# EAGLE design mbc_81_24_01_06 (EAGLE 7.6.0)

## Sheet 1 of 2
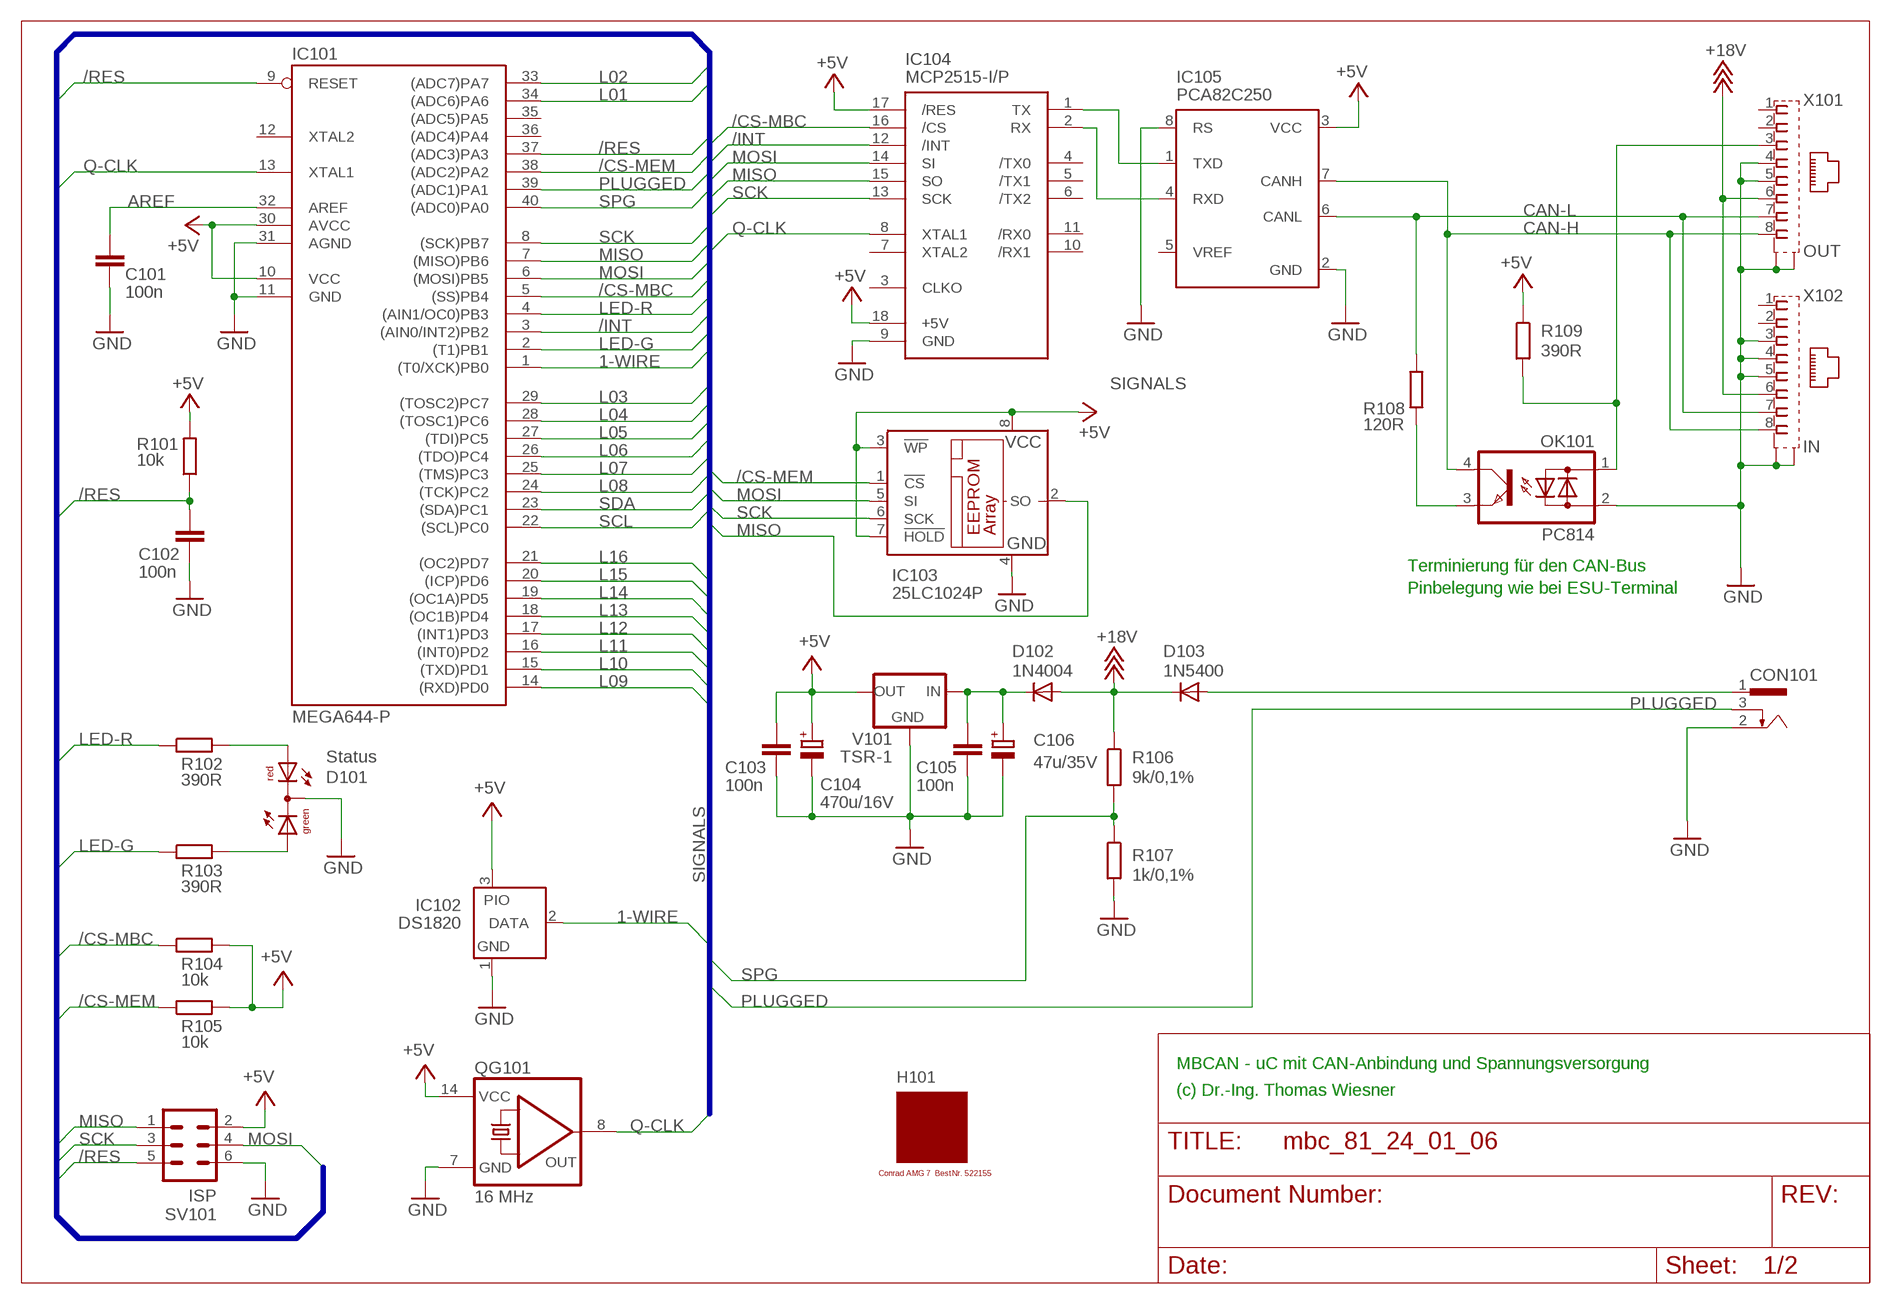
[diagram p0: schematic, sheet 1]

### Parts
C101  100n  C-EU025-025X050  [C025-025X050]
C102  100n  C-EU025-025X050  [C025-025X050]
C103  100n  C-EU025-025X050  [C025-025X050]
C104  470u/16V  CPOL-EUE3.5-8  [E3,5-8]
C105  100n  C-EU025-025X050  [C025-025X050]
C106  47u/35V  CPOL-EUE2.5-7  [E2,5-7]
CON101  POWER-JACK  [POWER-JACK]
D101  Status  DUOLED5MM  [DUOLED5MM]
D102  1N4004  [DO41-10]
D103  1N5400  [DO201-15]
H101  MODULGEHÄUSE-AMG-7  [MODULGEHÄUSE-1]
IC101  MEGA644-P  MEGA323-P  [DIL40]
IC102  DS1820  DS2405  [TO92-]
IC103  25LC1024P  25LC040P  [DIL8]
IC104  MCP2515-I/P  MCP2510-I/P  [DIL18]
IC105  PCA82C250  [DIL08]
OK101  PC814  [DIL04]
QG101  16 MHz  QG5860  [DIL14S]
R101  10k  R-EU_0207/10  [0207/10]
R102  390R  R-EU_0207/10  [0207/10]
R103  390R  R-EU_0207/10  [0207/10]
R104  10k  R-EU_0207/10  [0207/10]
R105  10k  R-EU_0207/10  [0207/10]
R106  9k/0,1%  R-EU_0207/10  [0207/10]
R107  1k/0,1%  R-EU_0207/10  [0207/10]
R108  120R  R-EU_0207/10  [0207/10]
R109  390R  R-EU_0207/10  [0207/10]
SV101  ISP  ML6  [ML6]
V101  TSR-1  [TRACO-TSR-1]
X101  OUT  0446200002  [0446200002]
X102  IN  0446200002  [0446200002]

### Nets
1-WIRE: IC101.1((T0/XCK)PB0) IC102.2(DATA)
+5V: C103.1 C104.+ IC101.10(VCC) IC101.30(AVCC) IC102.3(PIO) IC103.3(!WP) IC103.7(!HOLD) IC103.8(VCC) IC104.17(/RES) IC104.18(+5V) IC105.3(VCC) QG101.14(VCC) R101.2 R104.2 R105.2 R109.1 SV101.2 V101.OUT ; also sheet 2
+18V: D102.A D103.C R106.1 X101.6 X102.6
/CS-MBC: IC101.5((SS)PB4) IC104.16(/CS) R104.1
/CS-MEM: IC101.38((ADC2)PA2) IC103.1(!CS) R105.1
/INT: IC101.3((AIN0/INT2)PB2) IC104.12(/INT)
/RES: C102.1 IC101.9(RESET) IC101.37((ADC3)PA3) R101.1 SV101.5
AREF: C101.1 IC101.32(AREF)
CAN-H: IC105.7(CANH) OK101.4(C) X101.8 X102.8
CAN-L: IC105.6(CANL) R108.2 X101.7 X102.7
GND: C101.2 C102.2 C103.2 C104.- C105.2 C106.- CON101.2 D101.K(C) IC101.11(GND) IC101.31(AGND) IC102.1(GND) IC103.4(GND) IC104.9(GND) IC105.2(GND) IC105.8(RS) OK101.2(AC2) QG101.7(GND) R107.2 SV101.6 V101.GND X101.4 X101.5 X101.S@1(S1) X101.S@2(S2) X102.3 X102.4 X102.5 X102.S@1(S1) X102.S@2(S2) ; also sheet 2
L01: IC101.34((ADC6)PA6) ; also sheet 2
L02: IC101.33((ADC7)PA7) ; also sheet 2
L03: IC101.29((TOSC2)PC7) ; also sheet 2
L04: IC101.28((TOSC1)PC6) ; also sheet 2
L05: IC101.27((TDI)PC5) ; also sheet 2
L06: IC101.26((TDO)PC4) ; also sheet 2
L07: IC101.25((TMS)PC3) ; also sheet 2
L08: IC101.24((TCK)PC2) ; also sheet 2
L09: IC101.14((RXD)PD0) ; also sheet 2
L10: IC101.15((TXD)PD1) ; also sheet 2
L11: IC101.16((INT0)PD2) ; also sheet 2
L12: IC101.17((INT1)PD3) ; also sheet 2
L13: IC101.18((OC1B)PD4) ; also sheet 2
L14: IC101.19((OC1A)PD5) ; also sheet 2
L15: IC101.20((ICP)PD6) ; also sheet 2
L16: IC101.21((OC2)PD7) ; also sheet 2
LED-G: IC101.2((T1)PB1) R103.1
LED-R: IC101.4((AIN1/OC0)PB3) R102.1
MISO: IC101.7((MISO)PB6) IC103.2(SO) IC104.15(SO) SV101.1
MOSI: IC101.6((MOSI)PB5) IC103.5(SI) IC104.14(SI) SV101.4
N$1: IC104.1(TX) IC105.1(TXD)
N$2: IC104.2(RX) IC105.4(RXD)
N$3: OK101.3(E) R108.1
N$5: OK101.1(AC1) R109.2 X101.3
N$6: C105.1 C106.+ D102.C V101.IN
N$9: D101.AR R102.2
N$13: D101.AG R103.2
PLUGGED: CON101.3 IC101.39((ADC1)PA1)
Q-CLK: IC101.13(XTAL1) IC104.8(XTAL1) QG101.8(OUT)
SCK: IC101.8((SCK)PB7) IC103.6(SCK) IC104.13(SCK) SV101.3
SCL: IC101.22((SCL)PC0) ; also sheet 2
SDA: IC101.23((SDA)PC1) ; also sheet 2
SPG: IC101.40((ADC0)PA0) R106.2 R107.1
V-NETZTEIL1: CON101.1 D103.A
Unconnected: IC101.12(XTAL2) IC101.35((ADC5)PA5) IC101.36((ADC4)PA4) IC104.3(CLKO) IC104.4(/TX0) IC104.5(/TX1) IC104.6(/TX2) IC104.7(XTAL2) IC104.10(/RX1) IC104.11(/RX0) IC105.5(VREF) X101.1 X101.2 X102.1 X102.2

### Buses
SIGNALS

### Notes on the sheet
- Terminierung für den CAN-Bus
- Pinbelegung wie bei ESU-Terminal
- MBCAN - uC mit CAN-Anbindung und Spannungsversorgung
- (c) Dr.-Ing. Thomas Wiesner

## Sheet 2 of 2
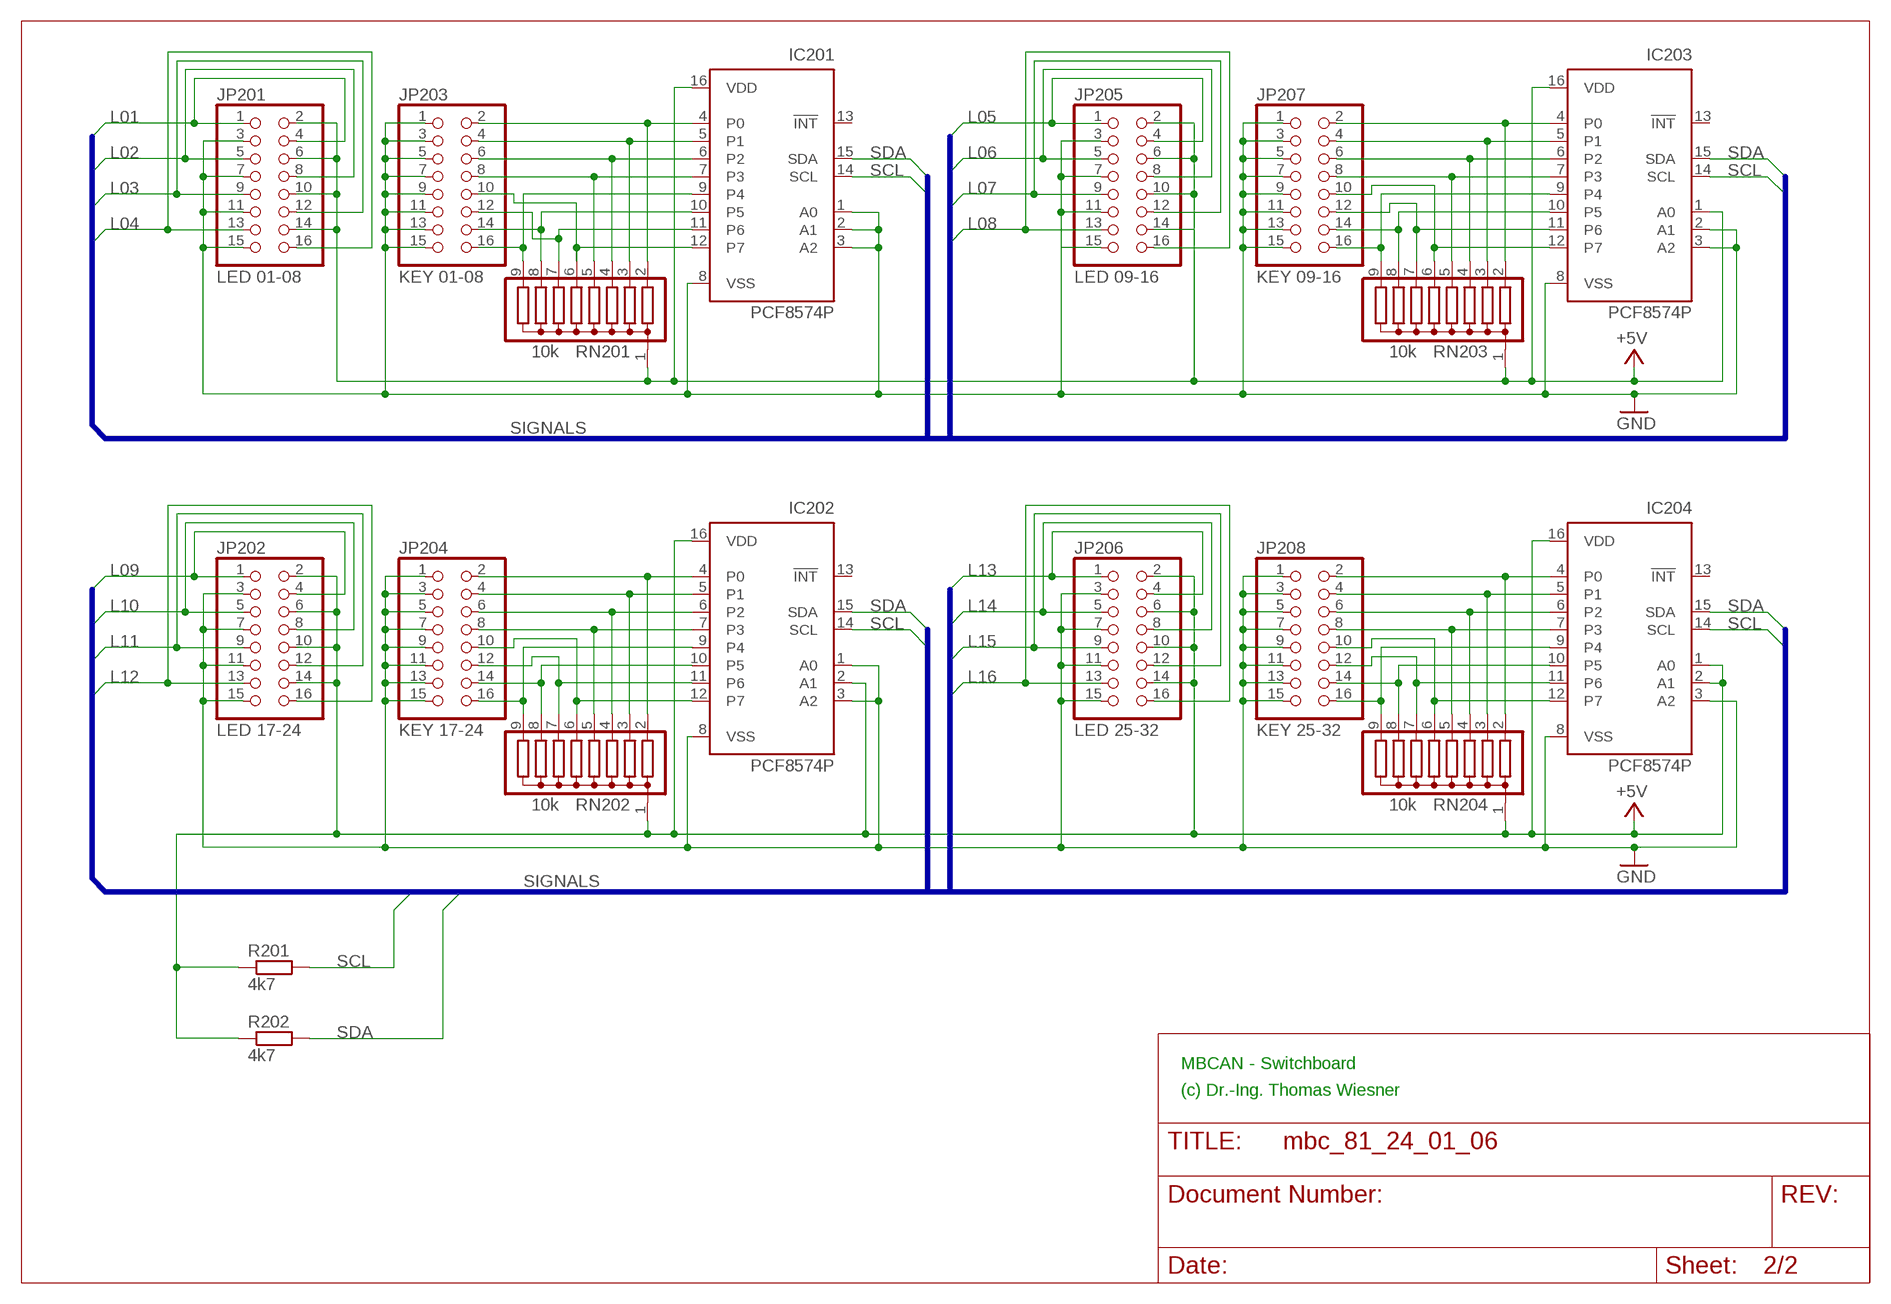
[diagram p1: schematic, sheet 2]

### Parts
IC201  PCF8574P  [DIL16]
IC202  PCF8574P  [DIL16]
IC203  PCF8574P  [DIL16]
IC204  PCF8574P  [DIL16]
JP201  LED 01-08  PINHD-2X8  [2X08]
JP202  LED 17-24  PINHD-2X8  [2X08]
JP203  KEY 01-08  PINHD-2X8  [2X08]
JP204  KEY 17-24  PINHD-2X8  [2X08]
JP205  LED 09-16  PINHD-2X8  [2X08]
JP206  LED 25-32  PINHD-2X8  [2X08]
JP207  KEY 09-16  PINHD-2X8  [2X08]
JP208  KEY 25-32  PINHD-2X8  [2X08]
R201  4k7  R-EU_0207/10  [0207/10]
R202  4k7  R-EU_0207/10  [0207/10]
RN201  10k  G08R  [SIL9]
RN202  10k  G08R  [SIL9]
RN203  10k  G08R  [SIL9]
RN204  10k  G08R  [SIL9]

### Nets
+5V: IC201.16(VDD) IC202.2(A1) IC202.16(VDD) IC203.1(A0) IC203.16(VDD) IC204.1(A0) IC204.2(A1) IC204.16(VDD) JP201.2 JP201.6 JP201.10 JP201.14 JP202.2 JP202.6 JP202.10 JP202.14 JP205.2 JP205.6 JP205.10 JP205.14 JP206.2 JP206.6 JP206.10 JP206.14 R201.1 R202.1 RN201.1 RN202.1 RN203.1 RN204.1 ; also sheet 1
GND: IC201.1(A0) IC201.2(A1) IC201.3(A2) IC201.8(VSS) IC202.1(A0) IC202.3(A2) IC202.8(VSS) IC203.2(A1) IC203.3(A2) IC203.8(VSS) IC204.3(A2) IC204.8(VSS) JP201.3 JP201.7 JP201.11 JP201.15 JP202.3 JP202.7 JP202.11 JP202.15 JP203.1 JP203.3 JP203.5 JP203.7 JP203.9 JP203.11 JP203.13 JP203.15 JP204.1 JP204.3 JP204.5 JP204.7 JP204.9 JP204.11 JP204.13 JP204.15 JP205.3 JP205.7 JP205.11 JP205.15 JP206.3 JP206.7 JP206.11 JP206.15 JP207.1 JP207.3 JP207.5 JP207.7 JP207.9 JP207.11 JP207.13 JP207.15 JP208.1 JP208.3 JP208.5 JP208.7 JP208.9 JP208.11 JP208.13 JP208.15 ; also sheet 1
L01: JP201.1 JP201.4 ; also sheet 1
L02: JP201.5 JP201.8 ; also sheet 1
L03: JP201.9 JP201.12 ; also sheet 1
L04: JP201.13 JP201.16 ; also sheet 1
L05: JP205.1 JP205.4 ; also sheet 1
L06: JP205.5 JP205.8 ; also sheet 1
L07: JP205.9 JP205.12 ; also sheet 1
L08: JP205.13 JP205.16 ; also sheet 1
L09: JP202.1 JP202.4 ; also sheet 1
L10: JP202.5 JP202.8 ; also sheet 1
L11: JP202.9 JP202.12 ; also sheet 1
L12: JP202.13 JP202.16 ; also sheet 1
L13: JP206.1 JP206.4 ; also sheet 1
L14: JP206.5 JP206.8 ; also sheet 1
L15: JP206.9 JP206.12 ; also sheet 1
L16: JP206.13 JP206.16 ; also sheet 1
N$15: IC202.4(P0) JP204.2 RN202.2
N$16: IC202.5(P1) JP204.4 RN202.3
N$17: IC202.6(P2) JP204.6 RN202.4
N$18: IC202.7(P3) JP204.8 RN202.5
N$19: IC202.12(P7) JP204.10 RN202.6
N$20: IC202.11(P6) JP204.12 RN202.7
N$21: IC202.10(P5) JP204.14 RN202.8
N$22: IC202.9(P4) JP204.16 RN202.9
N$23: IC201.4(P0) JP203.2 RN201.2
N$24: IC201.5(P1) JP203.4 RN201.3
N$25: IC201.6(P2) JP203.6 RN201.4
N$26: IC201.7(P3) JP203.8 RN201.5
N$27: IC201.9(P4) JP203.16 RN201.9
N$28: IC201.10(P5) JP203.14 RN201.8
N$29: IC201.11(P6) JP203.12 RN201.7
N$31: IC203.4(P0) JP207.2 RN203.2
N$32: IC203.5(P1) JP207.4 RN203.3
N$33: IC203.6(P2) JP207.6 RN203.4
N$34: IC203.7(P3) JP207.8 RN203.5
N$35: IC203.12(P7) JP207.10 RN203.6
N$36: IC203.11(P6) JP207.12 RN203.7
N$37: IC203.10(P5) JP207.14 RN203.8
N$38: IC203.9(P4) JP207.16 RN203.9
N$39: IC204.4(P0) JP208.2 RN204.2
N$40: IC204.5(P1) JP208.4 RN204.3
N$41: IC204.6(P2) JP208.6 RN204.4
N$42: IC204.7(P3) JP208.8 RN204.5
N$43: IC204.12(P7) JP208.10 RN204.6
N$44: IC204.11(P6) JP208.12 RN204.7
N$45: IC204.10(P5) JP208.14 RN204.8
N$46: IC204.9(P4) JP208.16 RN204.9
N$47: IC201.12(P7) JP203.10 RN201.6
SCL: IC201.14(SCL) IC202.14(SCL) IC203.14(SCL) IC204.14(SCL) R201.2 ; also sheet 1
SDA: IC201.15(SDA) IC202.15(SDA) IC203.15(SDA) IC204.15(SDA) R202.2 ; also sheet 1
Unconnected: IC201.13(!INT) IC202.13(!INT) IC203.13(!INT) IC204.13(!INT)

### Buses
SIGNALS

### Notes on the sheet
- MBCAN - Switchboard
- (c) Dr.-Ing. Thomas Wiesner

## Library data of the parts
C101-C103 C105 = rcl:C-EU: CAPACITOR, European symbol
C104 C106 = rcl:CPOL-EU: POLARIZED CAPACITOR, European symbol
CON101 = mbc:POWER-JACK
D101 = led:DUOLED5MM: DUO LED 2 colors, 5 mm, round
D102 = diode:1N4004: DIODE
D103 = diode:1N5400: DIODE
H101 = mbc:MODULGEHÄUSE-AMG-7: Gehäuse
IC101 = atmel:MEGA323-P: MICROCONTROLLER 32 Kbytes FLASH 2 Kbytes SRAM 1 Kbytes EEPROM USART 8-channel 10 bit ADC Source: avr.lbr; OC_FARNELL: unknown; OC_NEWARK: unknown
IC102 = maxim:DS2405: Addressable Switch DALLAS Semiconductor; MF: DALLAS SEMICONDUCTOR; MPN: DS2405; OC_FARNELL: 1188025; OC_NEWARK: 06F4645
IC103 = microchip:25*: Serial EEPROM 4K/ 8K , SPI bus; MF: MICROCHIP; MPN: 25LC040/P; OC_FARNELL: 9758100; OC_NEWARK: 96K4091
IC104 = mbc:MCP2510: BASIC-CAN 2.0a Controller Stand-alone CAN controller von Microchip
IC105 = micro-philips:PCA82C250: CAN CONTROLLER INTERFACE; OC_FARNELL: 3692358; OC_NEWARK: unknown
IC201-IC204 = micro-philips:PCF8574: I2C-Bus Remote 8-bit I/O expander http://www.semiconductors.philips.com/acrobat_download/datasheets/PCF8574_4.pdf; MPN: PCF8574PN; OC_FARNELL: 204020; OC_NEWARK: 11N8515
JP201-JP208 = pinhead:PINHD-2X8: PIN HEADER
OK101 = optocoupler:PC814: SHARP OPTO COUPLER; OC_FARNELL: 9707662; OC_NEWARK: unknown
QG101 = crystal:QG5860: CRYSTAL RESONATOR; OC_FARNELL: unknown; OC_NEWARK: unknown
R101-R109 = resistor:R-EU_: RESISTOR, European symbol
R201 R202 = rcl:R-EU_: RESISTOR, European symbol
RN201-RN204 = resistor-sil:G08R: SIL RESISTOR; OC_FARNELL: unknown; OC_NEWARK: unknown
SV101 = con-ml:ML6: HARTING; OC_FARNELL: unknown; OC_NEWARK: unknown
V101 = mbc:TSR-1: Spannungsregler Hersteller: TRACO Typ: TSR-1 5V: TSR 1-2450 Spg: 5V Strom: 1A Reichelt TSR 1-2450
X101 X102 = mbc:0446200002: RJ-45 INVERTED MODULAR JACK ASSEMBLY WITH RJ-11 KEEPOUT FEATURE Source: Data sheet MOLEX 0446200002 BUCHSE, RJ45, GESCHIRMT Source: Farnell; MF: MOLEX; MPN: 0446200002; OC_FARNELL: 9251910

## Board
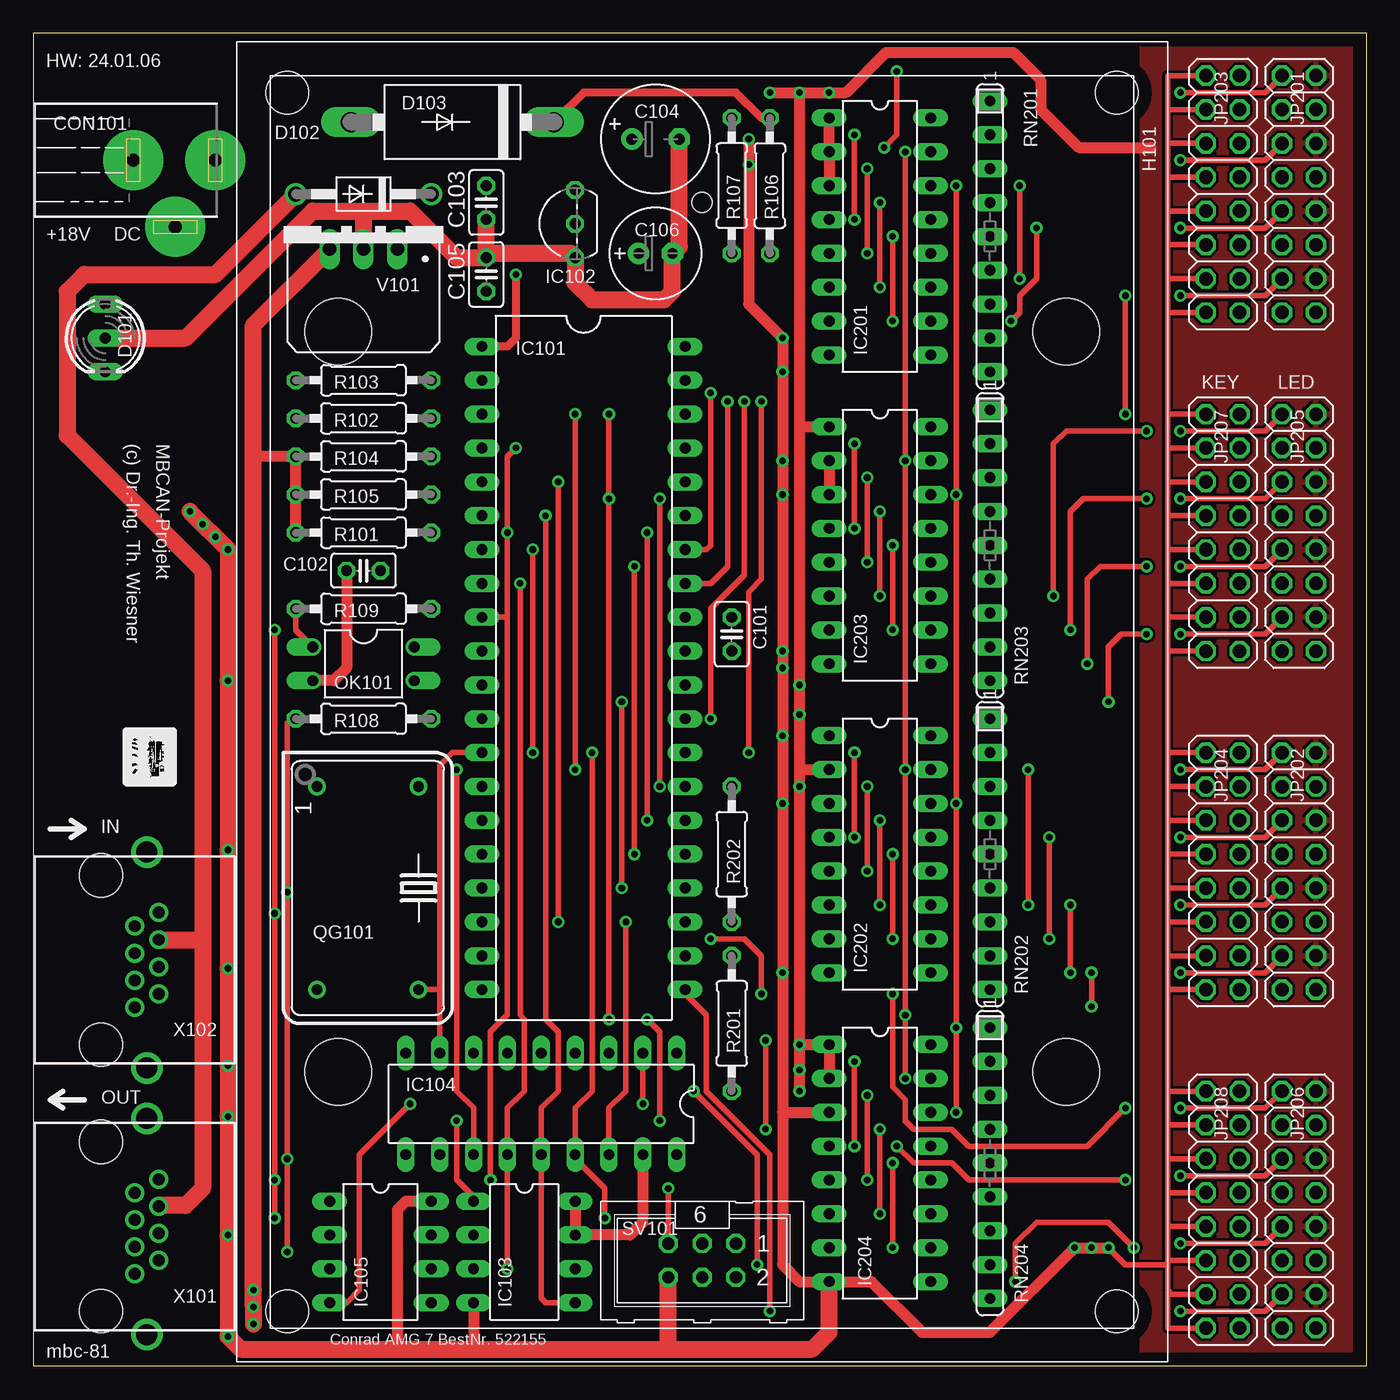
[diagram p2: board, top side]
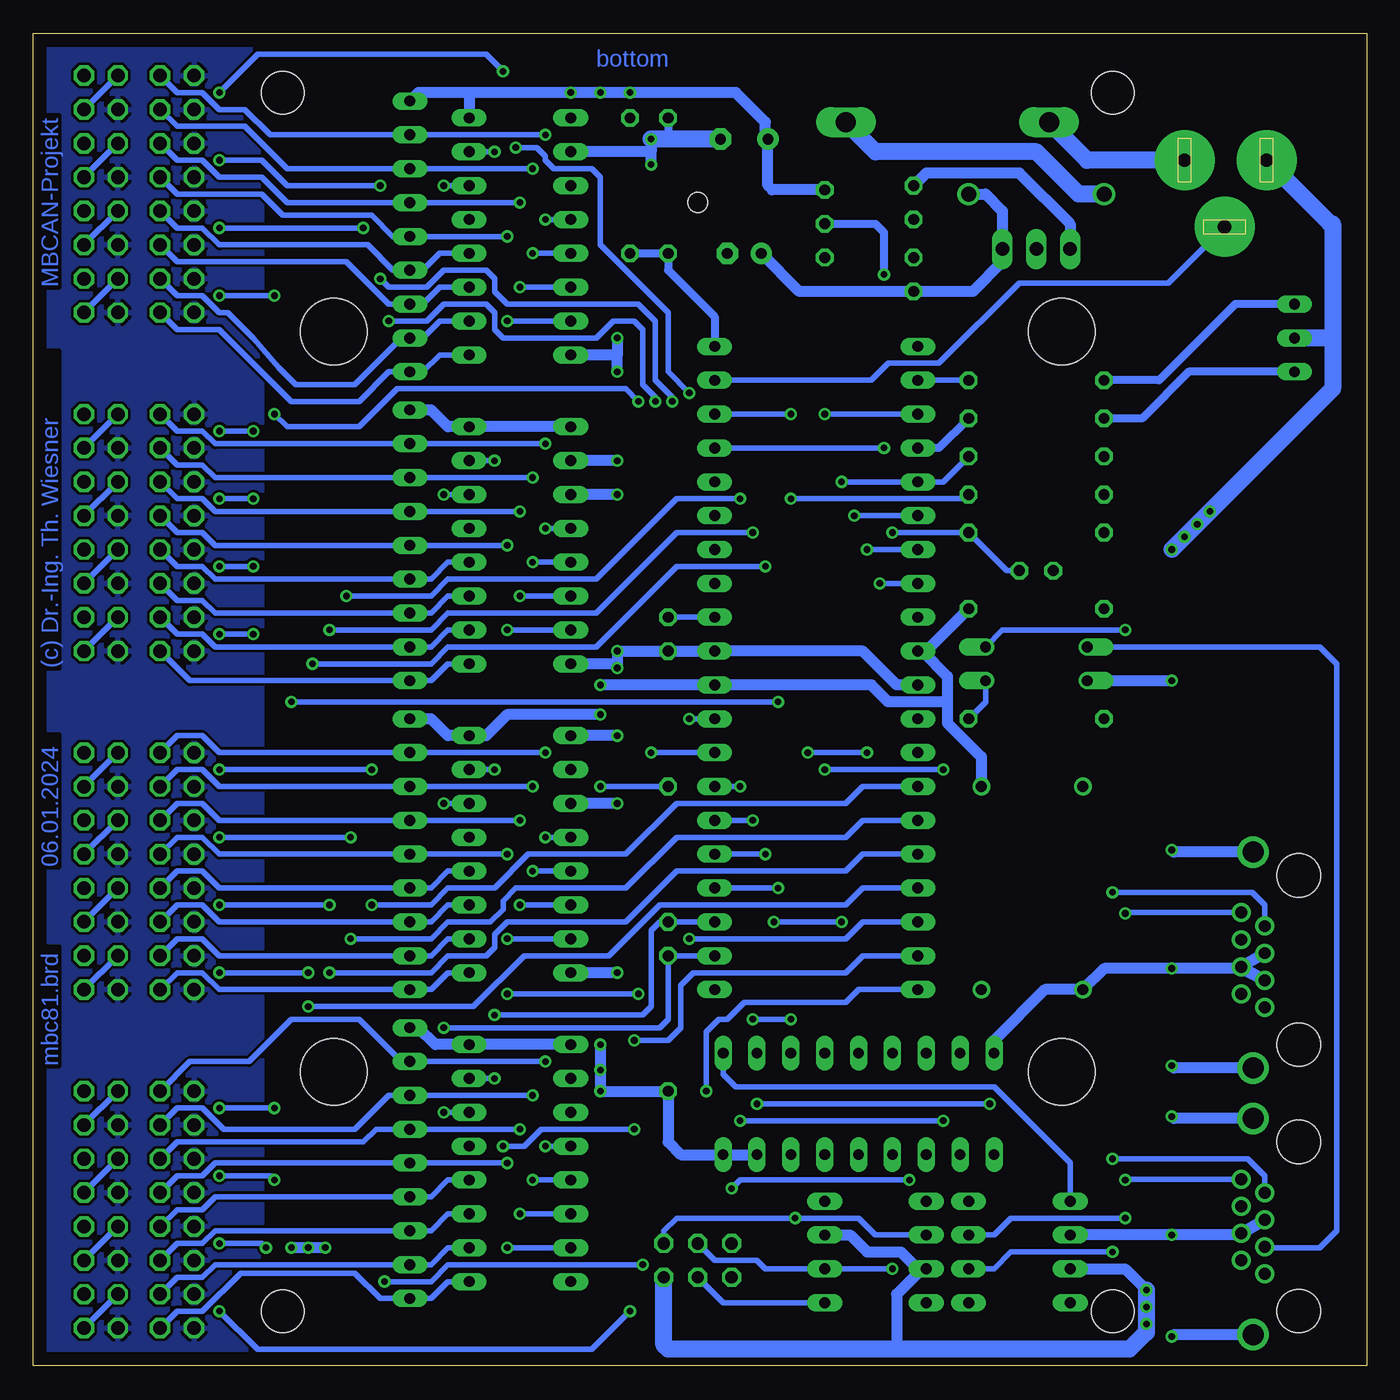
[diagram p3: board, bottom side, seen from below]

Size 100 x 99.99 mm. Coordinates in mm from the lower left corner, seen from the top.
Outline: 0,99.99 0,0 100,0 100,99.99 0,99.99
Copper layers (1*16): Top 0.035mm / dielectric 1.5mm / Bottom 0.035mm
Design rules "default *": minimum track width 10mil, minimum drill 0.5mm, track to track 8mil, track to pad 8mil, pad to pad 8mil, via to via 8mil, smd to smd 8mil, copper to edge 40mil, drill to drill 8mil, minimum pad ring 10mil, minimum via ring 8mil, stop-mask expansion 4mil, vias tented up to drill 0mil, thermal gap 10mil

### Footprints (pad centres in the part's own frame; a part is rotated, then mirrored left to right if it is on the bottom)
C025-025X050 = drill 0.813 octagon: 1 -1.27,0; 2 1.27,0
E3,5-8 = drill 0.813 pad 1.6: + -1.778,0 | drill 0.813 pad 1.6 octagon: - 1.778,0
E2,5-7 = drill 0.813 pad 1.6: + -1.27,0 | drill 0.813 pad 1.6 octagon: - 1.27,0
POWER-JACK = drill 1 pad 4.5: 1 0,6.03; 2 0,-0.12; 3 5,3.03
DUOLED5MM = drill 0.813 long: AG -2.54,0; AR 2.54,0; K 0,0
DO41-10 = drill 1.118: A 5.08,0; C -5.08,0
DO201-15 = drill 1.499 long: A 7.62,0; C -7.62,0
MODULGEHÄUSE-1 = hole 3.2: -45.72,-31.115; -45.72,31.115; 45.72,31.115; 45.72,-31.115 | hole 5: -27.781,-27.305; 27.781,-27.305; -27.781,27.305; 27.781,27.305 | hole 1.5: -37.465,0
DIL40 = drill 0.813 long: 1 -24.13,-7.62; 2 -21.59,-7.62; 3 -19.05,-7.62; 4 -16.51,-7.62; 5 -13.97,-7.62; 6 -11.43,-7.62; 7 -8.89,-7.62; 8 -6.35,-7.62; 9 -3.81,-7.62; 10 -1.27,-7.62; 11 1.27,-7.62; 12 3.81,-7.62; 13 6.35,-7.62; 14 8.89,-7.62; 15 11.43,-7.62; 16 13.97,-7.62; 17 16.51,-7.62; 18 19.05,-7.62; 19 21.59,-7.62; 20 24.13,-7.62; 21 24.13,7.62; 22 21.59,7.62; 23 19.05,7.62; 24 16.51,7.62; 25 13.97,7.62; 26 11.43,7.62; 27 8.89,7.62; 28 6.35,7.62; 29 3.81,7.62; 30 1.27,7.62; 31 -1.27,7.62; 32 -3.81,7.62; 33 -6.35,7.62; 34 -8.89,7.62; 35 -11.43,7.62; 36 -13.97,7.62; 37 -16.51,7.62; 38 -19.05,7.62; 39 -21.59,7.62; 40 -24.13,7.62
TO92- = drill 0.813 octagon: 1 -2.54,0; 2 0,0; 3 2.54,0
DIL8 = drill 0.813 long: 1 -3.81,-3.81; 2 -1.27,-3.81; 3 1.27,-3.81; 4 3.81,-3.81; 5 3.81,3.81; 6 1.27,3.81; 7 -1.27,3.81; 8 -3.81,3.81
DIL18 = drill 0.813 long: 1 -10.16,-3.81; 2 -7.62,-3.81; 3 -5.08,-3.81; 4 -2.54,-3.81 | drill 0.8 long: 5 0,-3.81; 6 2.54,-3.81; 7 5.08,-3.81; 8 7.62,-3.81; 9 10.16,-3.81; 10 10.16,3.81; 11 7.62,3.81; 12 5.08,3.81; 13 2.54,3.81; 14 0,3.81; 15 -2.54,3.81; 16 -5.08,3.81; 17 -7.62,3.81; 18 -10.16,3.81
DIL08 = drill 0.813 long: 1 -3.81,-3.81; 2 -1.27,-3.81; 3 1.27,-3.81; 4 3.81,-3.81; 5 3.81,3.81; 6 1.27,3.81; 7 -1.27,3.81; 8 -3.81,3.81
DIL16 = drill 0.813 long: 1 -8.89,-3.81; 2 -6.35,-3.81; 3 -3.81,-3.81; 4 -1.27,-3.81; 5 1.27,-3.81; 6 3.81,-3.81; 7 6.35,-3.81; 8 8.89,-3.81; 9 8.89,3.81; 10 6.35,3.81; 11 3.81,3.81; 12 1.27,3.81; 13 -1.27,3.81; 14 -3.81,3.81; 15 -6.35,3.81; 16 -8.89,3.81
2X08 = drill 1.016 octagon: 1 -8.89,-1.27; 2 -8.89,1.27; 3 -6.35,-1.27; 4 -6.35,1.27; 5 -3.81,-1.27; 6 -3.81,1.27; 7 -1.27,-1.27; 8 -1.27,1.27; 9 1.27,-1.27; 10 1.27,1.27; 11 3.81,-1.27; 12 3.81,1.27; 13 6.35,-1.27; 14 6.35,1.27; 15 8.89,-1.27; 16 8.89,1.27
DIL04 = drill 0.813 offset: 1 -1.27,-3.81; 2 1.27,-3.81; 3 1.27,3.81; 4 -1.27,3.81
DIL14S = drill 0.813: 1 -7.62,-3.81; 7 7.62,-3.81; 8 7.62,3.81; 14 -7.62,3.81
0207/10 = drill 0.813 octagon: 1 -5.08,0; 2 5.08,0
SIL9 = drill 0.813 long: 1 -10.16,0; 2 -7.62,0; 3 -5.08,0; 4 -2.54,0; 5 0,0; 6 2.54,0; 7 5.08,0; 8 7.62,0; 9 10.16,0
ML6 = drill 0.914 octagon: 1 -2.54,-1.27; 2 -2.54,1.27; 3 0,-1.27; 4 0,1.27; 5 2.54,-1.27; 6 2.54,1.27
TRACO-TSR-1 = drill 1.016 long: GND 0,2.54; IN -2.54,2.54; OUT 2.54,2.54
0446200002 = drill 0.889 pad 1.422: 1 3.556,2.54; 2 2.54,4.318; 3 1.524,2.54; 4 0.508,4.318; 5 -0.508,2.54; 6 -1.524,4.318; 7 -2.54,2.54; 8 -3.556,4.318 | drill 1.575 pad 2.286: S@1 -8.103,3.429; S@2 8.103,3.429 | hole 3.251: 6.35,0; -6.35,0

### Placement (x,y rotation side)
C101  52.39,54.91 270 top
C102  24.77,59.67 180 top
C103  33.97,87.29 270 top
C104  46.67,92.06 0 top
C105  33.97,81.9 90 top
C106  46.67,83.48 0 top
CON101  7.62,90.47 270 top
D101  5.4,77.13 270 top
D102  24.77,87.93 180 top
D103  31.43,93.33 180 top
H101  50.16,49.83 270 top
IC101  41.27,52.37 270 top
IC102  40.64,85.7 90 top
IC103  36.83,8.55 270 top
IC104  38.1,19.66 180 top
IC105  26.04,8.55 270 top
IC201  63.5,84.75 270 top
IC202  63.5,38.4 270 top
IC203  63.5,61.57 270 top
IC204  63.5,15.22 270 top
JP201  94.93,87.93 270 top
JP202  94.93,37.13 270 top
JP203  89.22,87.93 270 top
JP204  89.22,37.13 270 top
JP205  94.93,62.53 270 top
JP206  94.93,11.73 270 top
JP207  89.22,62.53 270 top
JP208  89.22,11.73 270 top
OK101  24.77,52.68 270 top
QG101  25.08,35.86 270 top
R101  24.77,62.53 180 top
R102  24.77,71.1 180 top
R103  24.77,73.96 180 top
R104  24.77,68.24 180 top
R105  24.77,65.39 180 top
R106  55.24,88.56 270 top
R107  52.39,88.56 90 top
R108  24.77,48.56 180 top
R109  24.77,56.81 180 top
R201  52.39,25.7 90 top
R202  52.39,38.4 270 top
RN201  71.75,84.75 270 top
RN202  71.75,38.4 270 top
RN203  71.75,61.57 270 top
RN204  71.75,15.22 270 top
SV101  50.16,7.92 180 top
V101  24.77,86.34 180 top
X101  5.08,10.46 270 top
X102  5.08,30.46 270 top

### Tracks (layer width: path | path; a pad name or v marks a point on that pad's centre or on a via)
1-WIRE  (via drill 0.5)
  Top 0.61: v36.2,81.9 36.2,77.13 35.56,76.5 IC101.1
  Bottom 0.61: IC102.2 36.83,85.7 36.2,85.07 v36.2,81.9
+5V  (via drill 0.5)
  Top 0.813: v57.47,95.55 v59.69,95.55 60.96,95.55 63.98,98.56 73.5,98.56 75.56,96.5 75.56,94.28 78.42,91.42 83.82,91.42 | v55.24,95.55 v57.47,95.55 | v57.47,95.55 57.47,70.47 | 57.47,70.47 v57.47,51.1 v57.47,48.88 57.47,44.75 | 57.47,44.75 v57.47,43.48 v57.47,24.11 | 57.47,70.47 IC203.1 | 57.47,44.75 IC202.2 | v57.47,24.11 IC204.1 IC204.2 | v57.47,24.11 v57.47,22.21 v57.47,20.62 | R101.2 R105.2 R104.2 16.51,68.24 | IC104.17 45.72,10.78 44.77,9.82 IC103.7 IC103.8
  Top 1.27: V101.OUT 16.51,78.09 16.51,68.24 v16.51,5.7 v16.51,4.43 v16.51,3.15
  Bottom 0.406: C104.+ 45.09,92.25 | v57.47,43.48 R202.1
  Bottom 0.813: IC104.17 IC104.18 51.44,15.86 52.39,16.81 R201.1 v57.47,20.62 v57.47,22.21 v57.47,24.11 | 33.34,53.64 31.43,51.73 31.43,49.83 | QG101.14 28.89,45.7 31.43,48.24 31.43,49.83 | IC102.3 44.58,88.25 44.9,88.56 C104.+ | V101.OUT 22.23,85.7 26.04,89.52 33.02,89.52 C103.1 | 45.09,92.25 45.09,93.33 47.31,95.55 v55.24,95.55 v57.47,95.55 v59.69,95.55 67.31,95.55 | 31.43,49.83 35.88,49.83 37.15,51.1 IC101.30 v57.47,51.1 | 67.31,95.55 71.12,95.55 RN201.1 | 67.31,95.55 IC201.16 | IC203.1 IC203.16 68.9,70.47 70.17,71.73 RN203.1 | RN202.1 70.17,48.56 68.9,47.29 IC202.16 66.04,47.29 64.45,48.88 v57.47,48.88 | RN204.1 71.12,25.38 69.85,24.11 IC204.16 IC204.1 | IC101.10 33.34,53.64 | 33.34,53.64 33.02,53.64 R109.1 | IC105.3 18.1,7.28 v16.51,5.7 | IC103.7 38.73,9.82 37.47,8.55 34.92,8.55 33.66,7.28 IC103.3 33.34,7.28 35.24,5.38 35.24,1.25
  Bottom 1.27: SV101.2 52.7,1.57 52.39,1.25 35.24,1.25 17.78,1.25 16.51,2.52 v16.51,3.15 v16.51,4.43 v16.51,5.7
  pour Top: 99.69,99.67 83.19,99.67 83.19,0.3 99.69,0.3
+18V
  Top 0.61: R106.1 54.61,93.64 52.7,95.55 41.27,95.55 D103.C
  Top 1.27: 12.7,32.05 12.7,59.67 2.54,69.83 2.54,80.62 3.81,81.9 13.65,81.9 D102.A | 12.7,32.05 12.7,13.32 11.43,12.04 9.46,12.04 X101.6 | X102.6 12.64,31.98 12.7,32.05
  Bottom 1.27: D102.A 21.59,87.93 24.77,91.1 36.83,91.1 D103.C
/CS-MBC  (via drill 0.5)
  Top 0.406: v39.37,66.34 v39.37,33.32 | v44.45,33.32 44.45,20.62 43.18,19.35 IC104.16
  Bottom 0.406: v39.37,66.34 IC101.5 31.75,66.34 R104.1 | v39.37,33.32 v44.45,33.32
/CS-MEM  (via drill 0.5)
  Top 0.406: v43.18,26.02 v43.18,65.07 v43.18,71.42 | IC103.1 33.02,12.68 31.75,13.95 v31.75,18.39 | v46.99,18.39 46.99,25.06 v46.04,26.02
  Bottom 0.406: v43.18,65.07 30.16,65.07 R105.1 | IC101.38 v43.18,71.42 | v31.75,18.39 v46.99,18.39 | v46.04,26.02 v43.18,26.02
/INT  (via drill 0.5)
  Top 0.406: IC104.12 33.02,19.35 31.75,20.62 v31.75,44.75 | v40.64,44.75 v40.64,71.42
  Bottom 0.406: v31.75,44.75 v40.64,44.75 | v40.64,71.42 IC101.3
/RES  (via drill 0.5)
  Top 0.406: 35.56,56.18 35.56,26.33 34.29,25.06 v34.29,13.95 | IC101.9 35.56,56.18 | 35.56,56.18 v35.56,62.53 35.56,68.24 v36.2,68.88 | v47.62,13.32 SV101.5
  Bottom 0.406: v36.2,68.88 IC101.37 | v35.56,62.53 R101.1 26.99,59.67 C102.1 | v34.29,13.95 46.99,13.95 v47.62,13.32
AREF
  Bottom 0.406: IC101.32 C101.1
CAN-H  (via drill 0.5)
  Top 0.406: v18.1,55.22 v18.1,33.95 v18.1,13.95 v18.1,11.09
  Bottom 0.406: X101.8 18.03,14.01 v18.1,13.95 | v18.1,55.22 27.3,55.22 OK101.4 | X102.8 18.03,34.02 v18.1,33.95 | v18.1,11.09 26.67,11.09 27.94,9.82 IC105.7
CAN-L  (via drill 0.5)
  Top 0.406: R108.2 19.37,48.56 19.05,48.24 v19.05,35.54 v19.05,15.54 v19.05,8.55
  Bottom 0.406: v19.05,8.55 26.67,8.55 27.94,7.28 IC105.6 | X101.7 7.62,14.27 8.89,15.54 v19.05,15.54 | X102.7 7.62,34.59 8.57,35.54 v19.05,35.54
GND  (via drill 0.5)
  Top 0.406: 85.09,94.28 85.09,96.82 JP203.1 | 85.09,91.74 85.09,94.28 | 85.09,89.2 85.09,91.74 | 85.09,86.66 85.09,89.2 | 85.09,84.12 85.09,86.66 | 85.09,81.58 85.09,84.12 | 85.09,79.04 85.09,81.58 | 85.09,94.28 JP203.3 | 85.09,91.74 JP203.5 | 85.09,89.2 JP203.7 | 85.09,86.66 JP203.9 | 85.09,84.12 JP203.11 | 85.09,81.58 JP203.13 | 85.09,79.04 JP203.15 | 85.09,71.42 85.09,79.04 | 85.09,68.88 85.09,71.42 | 85.09,66.34 85.09,68.88 | 85.09,63.8 85.09,66.34 | 85.09,61.26 85.09,63.8 | 85.09,58.72 85.09,61.26 | 85.09,56.18 85.09,58.72 | 85.09,53.64 85.09,56.18 | 85.09,46.02 85.09,53.64 | 85.09,43.48 85.09,46.02 | 85.09,40.94 85.09,43.48 | 85.09,38.4 85.09,40.94 | 85.09,35.86 85.09,38.4 | 85.09,33.32 85.09,35.86 | 85.09,30.78 85.09,33.32 | 85.09,28.24 85.09,30.78 | 85.09,20.62 85.09,28.24 | 85.09,18.08 85.09,20.62 | 85.09,15.54 85.09,18.08 | 85.09,13 85.09,15.54 | 85.09,10.46 85.09,13 | 85.09,7.6 85.09,5.7 | 85.09,5.7 85.09,2.84 JP208.15 | JP208.13 85.41,5.38 85.09,5.7 | 85.09,7.92 JP208.11 | 85.09,10.46 JP208.9 | 85.09,13 JP208.7 | 85.09,15.54 JP208.5 | 85.09,18.08 JP208.3 | 85.09,20.62 JP208.1 | 85.09,28.24 JP204.15 | 85.09,30.78 JP204.13 | 85.09,33.32 JP204.11 | 85.09,35.86 JP204.9 | 85.09,38.4 JP204.7 | 85.09,40.94 JP204.5 | 85.09,43.48 JP204.3 | 85.09,46.02 JP204.1 | 85.09,53.64 JP207.15 | 85.09,56.18 JP207.13 | 85.09,58.72 JP207.11 | 85.09,61.26 JP207.9 | 85.09,63.8 JP207.7 | 85.09,66.34 JP207.5 | 85.09,68.88 JP207.3 | 85.09,71.42 JP207.1 | 85.09,7.92 85.09,10.46 | v80.64,8.87 81.92,7.6 85.09,7.6 | 85.09,7.6 85.09,7.92 | v14.61,61.26 14.92,55.54
  Top 0.813: v53.66,92.06 v53.66,90.15 53.66,79.67 v56.2,77.13 v56.2,74.59 v56.2,67.92 v56.2,65.39 v56.2,53.64 v56.2,52.37 v56.2,47.29 v56.2,42.21 v56.2,29.51 56.2,19.03 | 56.2,19.03 56.2,7.6 57.47,6.33 IC204.8 62.87,6.33 66.67,2.52 71.75,2.52 v78.11,8.87 v79.38,8.87 v80.64,8.87 | 56.2,19.03 IC204.3 | IC201.1 IC201.2 IC201.3 | IC203.2 IC203.3 | C102.2 23.5,52.37 22.54,51.41 OK101.2 | IC105.8 27.94,12.36 27.3,11.73 27.3,1.25 | IC103.4 33.02,1.57 32.7,1.25
  Top 1.27: v11.75,64.12 v14.61,61.26 v14.61,51.41 v14.61,38.71 v14.61,29.82 v14.61,22.52 v14.61,18.71 v14.61,9.82 v14.61,2.2 15.56,1.25 27.3,1.25 32.7,1.25 47.62,1.25 | C104.- 48.45,83.99 C106.- 47.94,80.62 47.31,79.99 41.91,79.99 40.64,81.26 IC102.1 40.32,83.48 33.97,83.48 C105.2 | 24.77,86.66 V101.GND | 24.77,86.66 28.26,86.66 31.75,83.17 C105.2 | D101.K 11.43,77.13 20.95,86.66 24.77,86.66 | 47.62,1.25 SV101.6 | 47.62,1.25 58.42,1.25 59.69,2.52 IC204.8 | C105.2 C103.2
  Bottom 0.61: R107.2 52.39,92.37 52.7,92.06
  Bottom 0.813: IC101.11 35.24,51.1 37.78,53.64 IC101.31 C101.2 v56.2,53.64 56.2,52.68 | 53.66,91.1 IC201.2 | v53.66,92.06 53.66,91.1 | v53.66,90.15 53.66,91.1 | 56.2,75.86 IC201.8 | v56.2,77.13 56.2,75.86 | v56.2,74.59 56.2,75.86 | v56.2,67.92 IC203.2 | v56.2,65.39 IC203.3 | 56.2,52.68 IC203.8 | v56.2,52.37 56.2,52.68 | v56.2,47.29 IC202.1 | v56.2,42.21 IC202.3 | v56.2,29.51 IC202.8 | v80.64,8.87 v79.38,8.87 v78.11,8.87 | OK101.2 v14.61,51.41 | X102.S@1 14.45,38.56 v14.61,38.71 | X102.S@2 14.44,22.36 v14.61,22.52 | X101.S@1 14.45,18.56 v14.61,18.71 | X101.S@2 14.45,2.35 v14.61,2.2 | X102.5 X102.4 X102.3 9.53,29.82 v14.61,29.82 19.68,29.82 QG101.7 24.13,28.24 27.94,24.43 IC104.9 | X101.4 X101.5 9.53,9.82 v14.61,9.82 IC105.2
  Bottom 1.27: 2.54,77.13 2.54,85.7 2.74,85.7 CON101.2 | 2.54,77.13 D101.K | 2.54,77.13 2.54,73.32 v11.75,64.12 v12.7,63.16 v13.65,62.21 v14.61,61.26 | C104.- 52.7,92.06 v53.66,92.06
  pour Bottom: 99.69,99.67 82.87,99.67 82.87,0.3 99.69,0.3
L01  (via drill 0.5)
  Top 0.406: JP201.1 92.39,95.55 v86.04,95.55 | v64.77,97.14 64.77,92.37 v63.82,91.42 | v50.8,73.01 50.8,61.57 50.48,61.26 IC101.34
  Bottom 0.406: JP201.1 JP201.4 | v86.04,95.55 83.19,98.41 66.04,98.41 v64.77,97.14 | v63.82,91.42 62.23,91.42 61.59,90.79 61.59,90.47 60.96,89.83 58.1,89.83 57.47,89.2 57.47,84.12 52.39,79.04 52.39,74.59 v50.8,73.01
L02  (via drill 0.5)
  Top 0.406: JP201.5 92.39,90.47 v86.04,90.47 | v73.98,81.58 v73.98,88.56 | v52.07,72.37 52.07,59.99 50.8,58.72 IC101.33
  Bottom 0.406: JP201.5 JP201.8 | v86.04,90.47 82.87,90.47 80.96,88.56 v73.98,88.56 | v73.98,81.58 73.34,80.94 70.48,80.94 69.22,82.21 66.04,82.21 65.41,81.58 65.41,80.62 64.45,79.67 54.61,79.67 53.34,78.4 53.34,73.96 52.07,72.69 v52.07,72.37
L03  (via drill 0.5)
  Top 0.406: JP201.9 92.39,85.39 v86.04,85.39 | v75.25,85.39 75.25,81.58 73.98,80.31 73.98,79.04 v73.34,78.4 | v53.34,72.37 53.34,59.35 50.8,56.81 v50.8,48.56
  Bottom 0.406: JP201.9 JP201.12 | v75.25,85.39 v86.04,85.39 | v73.34,78.4 70.48,78.4 69.22,79.67 66.04,79.67 65.41,79.04 65.41,77.77 64.77,77.13 57.78,77.13 56.52,78.4 54.93,78.4 54.29,77.77 54.29,73.64 53.34,72.69 v53.34,72.37 | v50.8,48.56 IC101.29
L04  (via drill 0.5)
  Top 0.406: JP201.13 92.39,80.31 v86.04,80.31 | v81.92,71.42 v81.92,80.31 | v54.61,72.37 54.61,59.03 53.66,58.08 v53.66,46.02
  Bottom 0.406: JP201.13 JP201.16 | v81.92,80.31 v86.04,80.31 | v81.92,71.42 80.96,70.47 75.56,70.47 72.71,73.32 55.56,73.32 v54.61,72.37 | v53.66,46.02 IC101.28
L05  (via drill 0.5)
  Top 0.406: JP205.1 92.39,70.15 v86.04,70.15 | v46.99,65.07 v46.99,43.48 | v76.52,57.76 76.52,69.2 77.47,70.15 v83.5,70.15
  Bottom 0.406: JP205.1 JP205.4 | v46.99,43.48 IC101.27 | v46.99,65.07 51.75,65.07 57.78,59.03 68.9,59.03 70.17,57.76 v76.52,57.76 | v83.5,70.15 v86.04,70.15
L06  (via drill 0.5)
  Top 0.406: JP205.5 92.39,65.07 v86.04,65.07 | v83.5,65.07 78.74,65.07 77.79,64.12 v77.79,55.22 | v46.04,62.53 v46.04,40.94
  Bottom 0.406: JP205.5 JP205.8 | v83.5,65.07 v86.04,65.07 | v77.79,55.22 70.17,55.22 68.9,56.49 57.78,56.49 51.75,62.53 v46.04,62.53 | v46.04,40.94 IC101.26
L07  (via drill 0.5)
  Top 0.406: JP205.9 92.39,59.99 v86.04,59.99 | v83.5,59.99 80.01,59.99 79.06,59.03 v79.06,52.68 | v45.09,59.99 v45.09,38.4
  Bottom 0.406: JP205.9 JP205.12 | v83.5,59.99 v86.04,59.99 | v79.06,52.68 70.17,52.68 68.9,53.95 57.78,53.95 51.75,59.99 v45.09,59.99 | v45.09,38.4 IC101.25
L08  (via drill 0.5)
  Top 0.406: JP205.13 92.39,54.91 v86.04,54.91 | v83.5,54.91 81.6,54.91 80.64,53.95 v80.64,49.83 | v44.13,49.83 v44.13,35.86
  Bottom 0.406: JP205.13 JP205.16 | v83.5,54.91 v86.04,54.91 | v44.13,49.83 v80.64,49.83 | v44.13,35.86 IC101.24
L09  (via drill 0.5)
  Top 0.406: JP202.1 92.39,44.75 v86.04,44.75 | v74.61,34.59 v74.61,44.75
  Bottom 0.406: JP202.1 JP202.4 | v74.61,44.75 v86.04,44.75 | v74.61,34.59 70.17,34.59 68.9,35.86 65.41,35.86 62.87,38.4 55.56,38.4 51.75,42.21 39.05,42.21 37.78,43.48 IC101.14
L10  (via drill 0.5)
  Top 0.406: JP202.5 92.39,39.67 v86.04,39.67 | v76.2,32.05 v76.2,39.67
  Bottom 0.406: JP202.5 JP202.8 | v76.2,39.67 v86.04,39.67 | v76.2,32.05 70.17,32.05 68.9,33.32 65.72,33.32 64.77,34.27 64.77,34.9 63.82,35.86 55.56,35.86 51.75,39.67 39.05,39.67 37.78,40.94 IC101.15
L11  (via drill 0.5)
  Top 0.406: JP202.9 92.39,34.59 v86.04,34.59 | v77.79,29.51 v77.79,34.59
  Bottom 0.406: JP202.9 JP202.12 | v77.79,34.59 v86.04,34.59 | v77.79,29.51 70.17,29.51 68.9,30.78 66.04,30.78 65.41,31.41 65.41,32.36 64.45,33.32 55.56,33.32 51.75,37.13 39.05,37.13 37.78,38.4 IC101.16
L12  (via drill 0.5)
  Top 0.406: JP202.13 92.39,29.51 v86.04,29.51 | v79.38,26.97 v79.38,29.51
  Bottom 0.406: JP202.13 JP202.16 | v79.38,29.51 v86.04,29.51 | v79.38,26.97 66.99,26.97 63.18,30.78 56.83,30.78 53.02,34.59 39.05,34.59 37.78,35.86 IC101.17
L13  (via drill 0.5)
  Top 0.406: JP206.1 92.39,19.35 v86.04,19.35 | v50.8,32.05 53.34,32.05 54.61,30.78 v54.61,27.92 | v64.45,27.92 64.45,20.93 65.41,19.98 65.41,18.39 66.04,17.76 68.9,17.76 70.17,16.49 79.06,16.49 v81.92,19.35
  Bottom 0.406: JP206.1 JP206.4 | IC101.18 37.78,33.32 39.05,32.05 v50.8,32.05 | v54.61,27.92 v64.45,27.92 | v81.92,19.35 v86.04,19.35
L14  (via drill 0.5)
  Top 0.406: JP206.5 92.39,14.27 v86.04,14.27 | v54.93,24.43 v54.93,17.76 | v64.77,16.49 66.04,15.22 68.9,15.22 70.17,13.95 v81.92,13.95
  Bottom 0.406: JP206.5 JP206.8 | IC101.19 37.78,30.78 39.05,29.51 50.48,29.51 51.44,28.55 51.44,25.38 52.39,24.43 v54.93,24.43 | v54.93,17.76 61.91,17.76 63.18,16.49 v64.77,16.49 | v81.92,13.95 82.23,14.27 v86.04,14.27
L15  (via drill 0.5)
  Top 0.406: JP206.9 92.39,9.19 v86.04,9.19 | v49.53,20.62 54.29,15.86 v54.29,7.6 | v82.55,8.87 80.64,10.78 75.25,10.78 73.66,9.19 v73.66,6.33
  Bottom 0.406: JP206.9 JP206.12 | IC101.20 38.1,28.24 39.05,27.29 46.67,27.29 47.94,26.02 48.58,26.02 49.53,25.06 v49.53,20.62 | v54.29,7.6 68.9,7.6 70.17,6.33 v73.66,6.33 | v86.04,9.19 82.87,9.19 v82.55,8.87
L16  (via drill 0.5)
  Top 0.406: JP206.13 92.39,4.11 v86.04,4.11 | IC101.21 48.9,27.92 50.48,26.33 50.48,20.62 55.24,15.86 v55.24,4.11
  Bottom 0.406: JP206.13 JP206.16 | v55.24,4.11 58.1,1.25 83.19,1.25 v86.04,4.11
LED-G
  Bottom 0.406: IC101.2 R103.1
LED-R
  Bottom 0.61: IC101.4 32.07,68.88 R102.1
MISO  (via drill 0.5)
  Top 0.406: v37.47,61.26 v37.47,46.02 | v41.91,46.02 41.91,20.62 40.64,19.35 IC104.15 40.64,15.54 42.86,13.32 v42.86,11.09
  Bottom 0.406: IC101.7 v37.47,61.26 | v37.47,46.02 v41.91,46.02 | SV101.1 52.7,10.14 51.75,11.09 v42.86,11.09 38.1,11.09 36.83,9.82 IC103.2
MOSI  (via drill 0.5)
  Top 0.406: v38.42,63.8 38.42,26.02 39.37,25.06 39.37,20.62 38.1,19.35 IC104.14 38.1,5.06 38.42,4.74 IC103.5
  Bottom 0.406: IC101.6 v38.42,63.8 | IC103.5 48.26,4.74 SV101.4
N$1
  Bottom 0.406: IC105.1 22.23,15.22 27.94,20.93 47.31,20.93 48.26,21.89 IC104.1
N$2  (via drill 0.5)
  Top 0.406: IC105.4 23.5,4.74 24.45,5.7 24.45,15.86 v28.26,19.66 | v45.72,19.66 IC104.2
  Bottom 0.406: v28.26,19.66 v45.72,19.66
N$3
  Bottom 0.406: OK101.3 28.57,49.83 R108.1
N$5
  Top 0.406: R109.2 19.68,55.22 OK101.1
  Bottom 0.406: OK101.1 3.49,53.95 2.22,52.68 2.22,10.14 3.49,8.87 7.56,8.87 X101.3
N$6
  Bottom 0.813: D102.C 28.57,87.93 27.3,86.66 V101.IN 27.3,82.85 29.53,80.62 C105.1 42.55,80.62 C106.+
N$9
  Bottom 0.61: R102.2 16.83,71.1 13.34,74.59 D101.AR
N$13
  Bottom 0.61: R103.2 15.56,73.96 9.84,79.67 D101.AG
N$15  (via drill 0.5)
  Top 0.406: v61.59,46.02 v61.59,39.67
  Bottom 0.406: JP204.2 89.22,47.29 87.31,47.29 86.04,46.02 RN202.2 v61.59,46.02 | v61.59,39.67 IC202.4
N$16  (via drill 0.5)
  Top 0.406: v62.55,43.48 v62.55,37.13
  Bottom 0.406: JP204.4 89.22,44.75 87.31,44.75 86.04,43.48 RN202.3 v62.55,43.48 | v62.55,37.13 IC202.5
N$17  (via drill 0.5)
  Top 0.406: v63.5,34.59 v63.5,40.94
  Bottom 0.406: JP204.6 89.22,42.21 87.31,42.21 86.04,40.94 RN202.4 v63.5,40.94 | IC202.6 v63.5,34.59
N$18  (via drill 0.5)
  Top 0.406: v64.45,32.05 v64.45,38.4
  Bottom 0.406: JP204.8 89.22,39.67 87.31,39.67 86.04,38.4 RN202.5 v64.45,38.4 | IC202.7 v64.45,32.05
N$19
  Bottom 0.406: JP204.10 89.22,37.13 87.31,37.13 86.04,35.86 RN202.6 70.17,35.86 68.9,37.13 IC202.12
N$20
  Bottom 0.406: JP204.12 89.22,34.59 87.31,34.59 86.04,33.32 RN202.7 70.17,33.32 68.9,34.59 IC202.11
N$21
  Bottom 0.406: JP204.14 89.22,32.05 87.31,32.05 86.04,30.78 RN202.8 70.17,30.78 68.9,32.05 IC202.10
N$22
  Bottom 0.406: JP204.16 89.22,29.51 87.31,29.51 86.04,28.24 RN202.9 70.17,28.24 68.9,29.51 IC202.9
N$23  (via drill 0.5)
  Top 0.406: v61.59,92.37 v61.59,86.02
  Bottom 0.406: JP203.2 89.22,95.55 87.31,95.55 86.04,94.28 84.14,94.28 82.23,92.37 RN201.2 v61.59,92.37 | v61.59,86.02 IC201.4
N$24  (via drill 0.5)
  Top 0.406: v62.55,89.83 v62.55,83.48
  Bottom 0.406: JP203.4 89.22,93.01 84.14,93.01 80.96,89.83 RN201.3 v62.55,89.83 | v62.55,83.48 IC201.5
N$25  (via drill 0.5)
  Top 0.406: v63.5,80.94 v63.5,87.29
  Bottom 0.406: JP203.6 89.22,90.47 87.31,90.47 86.04,89.2 82.87,89.2 80.96,87.29 RN201.4 v63.5,87.29 | IC201.6 v63.5,80.94
N$26  (via drill 0.5)
  Top 0.406: v64.45,78.4 v64.45,84.75
  Bottom 0.406: JP203.8 89.22,87.93 82.87,87.93 81.28,86.34 74.61,86.34 73.03,84.75 RN201.5 v64.45,84.75 | IC201.7 v64.45,78.4
N$27
  Bottom 0.406: JP203.16 89.22,77.77 86.04,77.77 80.64,72.37 75.56,72.37 73.34,74.59 RN201.9 70.8,74.59 69.53,75.86 IC201.9
N$28
  Bottom 0.406: JP203.14 89.22,80.31 87.31,80.31 86.04,79.04 85.41,79.04 83.5,77.13 81.6,74.91 80.33,73.64 75.88,73.64 72.39,77.13 RN201.8 70.8,77.13 69.53,78.4 IC201.10
N$29
  Bottom 0.406: JP203.12 89.22,82.85 76.52,82.85 73.34,79.67 RN201.7 70.8,79.67 69.53,80.94 IC201.11
N$31  (via drill 0.5)
  Top 0.406: v61.59,69.2 v61.59,62.84
  Bottom 0.406: JP207.2 89.22,70.15 87.31,70.15 86.36,69.2 RN203.2 v61.59,69.2 | v61.59,62.84 IC203.4
N$32  (via drill 0.5)
  Top 0.406: v62.55,66.66 v62.55,60.3
  Bottom 0.406: JP207.4 89.22,67.61 87.31,67.61 86.36,66.66 RN203.3 v62.55,66.66 | v62.55,60.3 IC203.5
N$33  (via drill 0.5)
  Top 0.406: v63.5,57.76 v63.5,64.12
  Bottom 0.406: JP207.6 89.22,65.07 87.31,65.07 86.36,64.12 RN203.4 v63.5,64.12 | IC203.6 v63.5,57.76
N$34  (via drill 0.5)
  Top 0.406: v64.45,55.22 v64.45,61.57
  Bottom 0.406: JP207.8 89.22,62.53 87.31,62.53 86.36,61.57 RN203.5 v64.45,61.57 | IC203.7 v64.45,55.22
N$35
  Bottom 0.406: JP207.10 89.22,59.99 87.31,59.99 86.36,59.03 RN203.6 70.17,59.03 68.9,60.3 IC203.12
N$36
  Bottom 0.406: JP207.12 89.22,57.45 87.31,57.45 86.36,56.49 RN203.7 70.17,56.49 68.9,57.76 IC203.11
N$37
  Bottom 0.406: JP207.14 89.22,54.91 87.31,54.91 86.36,53.95 RN203.8 70.17,53.95 68.9,55.22 IC203.10
N$38
  Bottom 0.406: JP207.16 88.27,51.41 RN203.9 70.17,51.41 68.9,52.68 IC203.9
N$39  (via drill 0.5)
  Top 0.406: v61.59,22.84 v61.59,16.49
  Bottom 0.406: JP208.2 88.27,22.84 83.82,22.84 80.64,26.02 75.56,26.02 72.39,22.84 RN204.2 v61.59,22.84 | v61.59,16.49 IC204.4
N$40  (via drill 0.5)
  Top 0.406: v62.55,20.3 v62.55,13.95
  Bottom 0.406: JP208.4 89.22,19.35 87.31,19.35 85.72,17.76 75.88,17.76 73.34,20.3 RN204.3 v62.55,20.3 | v62.55,13.95 IC204.5
N$41  (via drill 0.5)
  Top 0.406: v63.5,11.41 v63.5,17.76
  Bottom 0.406: JP208.6 89.22,16.81 75.25,16.81 74.3,17.76 RN204.4 v63.5,17.76 | IC204.6 v63.5,11.41
N$42  (via drill 0.5)
  Top 0.406: v64.45,8.87 v64.45,15.22
  Bottom 0.406: JP208.8 89.22,14.27 87.31,14.27 86.36,15.22 RN204.5 v64.45,15.22 | IC204.7 v64.45,8.87
N$43
  Bottom 0.406: JP208.10 89.22,11.73 87.31,11.73 86.36,12.68 RN204.6 70.17,12.68 68.9,13.95 IC204.12
N$44
  Bottom 0.406: JP208.12 89.22,9.19 87.31,9.19 86.36,10.14 RN204.7 70.17,10.14 68.9,11.41 IC204.11
N$45
  Bottom 0.406: JP208.14 89.22,6.65 87.31,6.65 86.36,7.6 RN204.8 70.17,7.6 68.9,8.87 IC204.10
N$46
  Bottom 0.406: JP208.16 89.22,4.11 87.31,4.11 84.45,6.97 75.88,6.97 73.98,5.06 RN204.9 70.17,5.06 68.9,6.33 IC204.9
N$47
  Bottom 0.406: JP203.10 89.22,85.39 87.31,85.39 86.04,84.12 74.93,84.12 73.03,82.21 RN201.6 70.8,82.21 69.53,83.48 IC201.12
PLUGGED
  Bottom 0.406: IC101.39 37.15,73.96 35.88,75.23 32.07,75.23 26.04,81.26 14.86,81.26 CON101.3
Q-CLK
  Top 0.406: IC101.13 31.43,46.02 30.48,45.06 30.48,28.24 | 30.48,28.24 IC104.8 | 30.48,28.24 QG101.8
SCK  (via drill 0.5)
  Top 0.406: v36.51,58.72 36.51,26.33 36.83,26.02 36.83,20.62 35.56,19.35 IC104.13 v35.56,7.28
  Bottom 0.406: IC101.8 v36.51,58.72 | SV101.3 48.9,7.92 45.72,7.92 45.09,7.28 IC103.6 v35.56,7.28
SCL  (via drill 0.5)
  Top 0.406: v69.22,88.56 v69.22,65.39 v69.22,42.21 v69.22,25.38 v69.22,19.03
  Bottom 0.406: IC201.14 v69.22,88.56 | v69.22,19.03 IC204.14 | v69.22,65.39 IC203.14 | v69.22,42.21 IC202.14 | v69.22,25.38 53.02,25.38 52.39,26.02 R201.2 IC101.22
SDA  (via drill 0.5)
  Top 0.406: v65.41,91.1 v65.41,67.92 v65.41,44.75 v65.41,26.33 v65.41,21.57
  Bottom 0.406: v65.41,91.1 IC201.15 | v65.41,21.57 IC204.15 | v65.41,44.75 IC202.15 | v65.41,67.92 IC203.15 | IC101.23 R202.2 53.02,33.32 53.66,32.68 53.66,26.97 54.29,26.33 v65.41,26.33
SPG
  Bottom 0.61: R106.2 R107.1 52.39,82.21 48.9,78.72 IC101.40
V-NETZTEIL1
  Bottom 1.27: CON101.1 20.95,90.47 D103.A

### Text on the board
Bottom: bottom | MBCAN-Projekt | (c) Dr.-Ing. Th. Wiesner | 06.01.2024 | mbc81.brd
tNames: HW: 24.01.06 | +18V | DC | KEY | LED | (c) Dr.-Ing. Th. Wiesner | MBCAN-Projekt | IN | OUT | mbc-81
